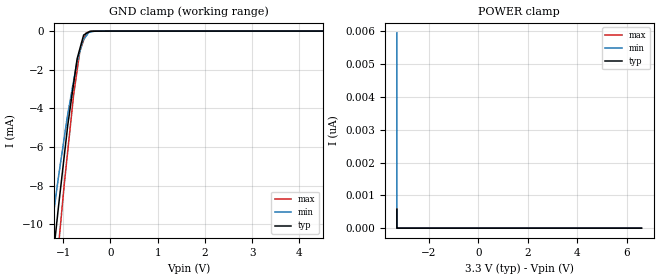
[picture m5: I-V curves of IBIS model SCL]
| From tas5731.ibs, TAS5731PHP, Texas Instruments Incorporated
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[Model]   SCL
Model_type   Input
Vinl = .8
Vinh = 2
|   typ   min   max
C_comp   0.7443p   0.7440p   0.7473p
[Voltage Range]   3.3   3   3.6
[Temperature Range]   27   125   0
[Power Clamp Reference]   3.3   3   3.6
[GND Clamp Reference]   -0   -0   -0
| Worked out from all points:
|   GND clamp passes 1 mA (typ) near -0.66 V on its own axis
[GND Clamp]
|   Voltage   I(typ)   I(min)   I(max)
-3.3V     -1.514A    -1.356A    -1.56A
-1.372V   -15.31mA   -12.42mA   -18.38mA
-1.237V   -12.18mA   -9.983mA   -14.75mA
-1.157V   -10.35mA   -8.537mA   -12.59mA
-1.102V   -9.096mA   -7.552mA   -11.15mA
-904.1mV  -4.85mA    -4.296mA   -6.176mA
-780.4mV  -2.711mA   -2.57mA    -3.29mA
-706.1mV  -1.425mA   -1.591mA   -2.019mA
-648.3mV  -913.9uA   -1.062mA   -1.032mA
-516.3mV  -130.2uA   -261uA     -91.17uA
-320.4mV  -5.141uA   -2.758uA   -960.6nA
6.6V      0A         0A         0A
[POWER Clamp]
|   Voltage   I(typ)   I(min)   I(max)
-3.3V     572.5pA    5.955nA    588.9pA
-3.3V     0A         0A         0A
-3.3V     0A         0A         0A
6.6V      0A         0A         0A
